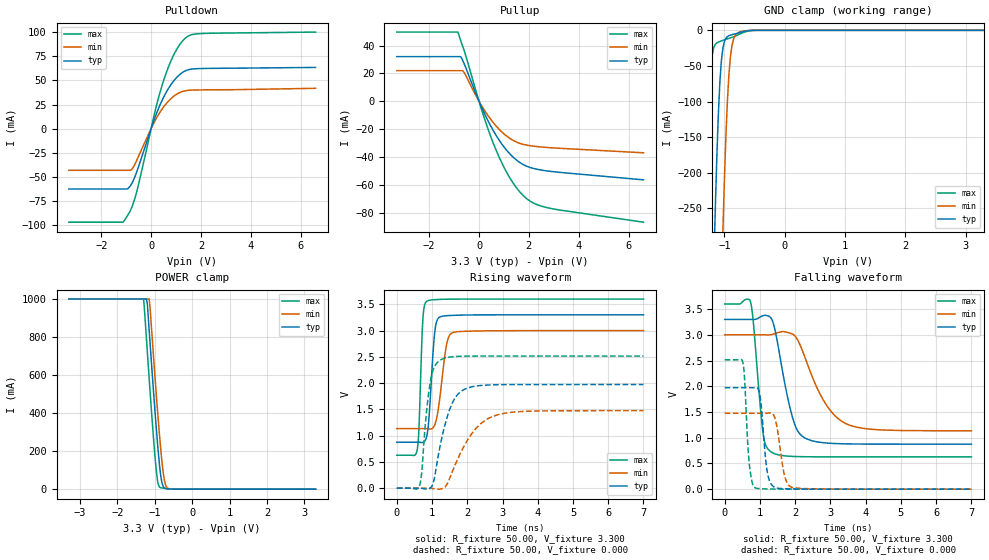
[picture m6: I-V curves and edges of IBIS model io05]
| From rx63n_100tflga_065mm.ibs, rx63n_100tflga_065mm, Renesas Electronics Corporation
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[Model]   io05
Model_type   I/O
Polarity   Non-Inverting
Enable   Active-High
Vinl  =   0.660V
Vinh  =   2.640V
Vmeas =   1.650V
Cref  =   30.00pF
| variable   typ   min   max
C_comp   3.770pF   3.770pF   3.770pF
| variable   typ   min   max
[Temperature Range]   45.000   105.000   -40.000
| variable   typ   min   max
[Voltage Range]   3.300V   3.000V   3.600V
| variable   typ   min   max
[Pullup Reference]   3.300V   3.000V   3.600V
| variable   typ   min   max
[Pulldown Reference]   0.000V   0.000V   0.000V
| variable   typ   min   max
[POWER Clamp Reference] 3.300V   3.000V   3.600V
| variable   typ   min   max
[GND Clamp Reference]   0.000V   0.000V   0.000V
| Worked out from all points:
|   slope of the pulldown table from 0 to 0.495 V, typ, clamps not added: 15.4 ohm
|   slope of the pullup table from 0 to 0.495 V, typ, clamps not added: 26.5 ohm
|   GND clamp passes 1 mA (typ) near -0.64 V on its own axis
|   POWER clamp passes 1 mA (typ) near -0.59 V on its own axis
|   rising waveform, R_fixture 50.00, V_fixture 3.300: 20-80 % time 140ps typ, 208ps min, 90.5ps max; typ from 0.875 V to 3.3 V
|   rising waveform, R_fixture 50.00, V_fixture 0.000: 20-80 % time 428ps typ, 745ps min, 217ps max; typ from 0 V to 1.97 V
|   falling waveform, R_fixture 50.00, V_fixture 3.300: 20-80 % time 432ps typ, 781ps min, 221ps max; typ from 3.3 V to 0.875 V
|   falling waveform, R_fixture 50.00, V_fixture 0.000: 20-80 % time 154ps typ, 198ps min, 122ps max; typ from 1.97 V to 0 V
[Pulldown]
| io05_strong Pulldown rx631_rx63n
| Thu Mar 22 17:15:49 2012
| voltage   I(typ)   I(min)   I(max)
-3.3V     -62.62mA   -43.25mA   -97.14mA
-1.15V    -62.62mA   -43.25mA   -97.14mA
-1.025V   -62.62mA   -43.25mA   -93.52mA
-800mV    -58.13mA   -42.94mA   -83.32mA
-600mV    -46.6mA    -34.2mA    -67.76mA
175mV     12.96mA    9.062mA    19.78mA
525mV     33.78mA    23.32mA    51.76mA
950mV     50.91mA    34.42mA    78.65mA
1.4V      60.32mA    39.47mA    94.53mA
1.7V      62.04mA    40.07mA    97.97mA
2.1V      62.47mA    40.25mA    98.84mA
6.6V      63.56mA    41.89mA    100.3mA
[Pullup]
| io05_strong Pullup rx631_rx63n
| Thu Mar 22 17:15:49 2012
| voltage   I(typ)   I(min)   I(max)
-3.3V     32.05mA    21.95mA    49.68mA
-850mV    32.05mA    21.95mA    49.68mA
-725mV    31.77mA    21.95mA    43.08mA
-625mV    28.07mA    21.43mA    37.88mA
175mV     -7.149mA   -5.281mA   -10.11mA
700mV     -24.99mA   -18.1mA    -35.76mA
1V        -32.82mA   -23.46mA   -47.4mA
1.325V    -39.44mA   -27.7mA    -57.61mA
1.95V     -46.99mA   -31.69mA   -70.56mA
2.3V      -48.81mA   -32.55mA   -74.14mA
2.9V      -50.5mA    -33.47mA   -77.15mA
6.6V      -56.53mA   -37.08mA   -86.96mA
[GND Clamp]
| io05_strong GNDClamp rx631_rx63n
| Thu Mar 22 17:15:49 2012
| voltage   I(typ)   I(min)   I(max)
-3.3V     -1A        -1A        -1A
-1.325V   -916.3mA   -1A        -321.6mA
-1.225V   -508.3mA   -1A        -56.05mA
-1.175V   -327.1mA   -831.8mA   -23.6mA
-1.15V    -246.5mA   -730.6mA   -19.51mA
-1.075V   -71.99mA   -445.9mA   -15.62mA
-1.025V   -24.89mA   -280.5mA   -14.09mA
-975mV    -11.12mA   -147.9mA   -12.65mA
-925mV    -7.484mA   -61.53mA   -11.26mA
-850mV    -5.559mA   -12.59mA   -9.146mA
-675mV    -1.555mA   -930uA     -2.738mA
3.3V      0A         0A         0A
[POWER Clamp]
| io05_strong PWRClamp rx631_rx63n
| Thu Mar 22 17:15:49 2012
| voltage   I(typ)   I(min)   I(max)
-3.3V     1A         1A         1A
-1.3V     1A         1A         1A
-1.225V   1A         1A         792.2mA
-1.2V     974.1mA    1A         720.1mA
-1.15V    831.4mA    1A         577.8mA
-975mV    355.2mA    535.2mA    125.1mA
-925mV    233.2mA    405.8mA    41.42mA
-875mV    126.6mA    283.8mA    11.35mA
-825mV    49.1mA     174.1mA    7.014mA
-750mV    7.224mA    53.11mA    4.912mA
-625mV    1.442mA    2.321mA    1.9mA
3.3V      0A         0A         0A
[Ramp]
dV/dt_r   1.184/427.74p  0.886/744.56p  1.509/216.62p
dV/dt_f   1.455/431.05p  1.119/780.77p  1.783/220.80p
R_load = 50.00ohm
[Rising Waveform]
| io05_strong Rising-High rx631_rx63n
| Thu Mar 22 17:15:49 2012
R_fixture = 50.00
V_fixture = 3.300
V_fixture_min = 3.000
V_fixture_max = 3.600
C_fixture = 0.00pF
| Time   V(typ)   V(min)   V(max)
0s        875mV      1.135V     628mV
575ps     876mV      1.135V     718mV
630ps     875mV      1.135V     1.161V
740ps     871mV      1.136V     3.21V
855ps     1.006V     1.133V     3.56V
1.075ns   2.955V     1.203V     3.588V
1.22ns    3.258V     1.714V     3.594V
1.415ns   3.283V     2.737V     3.597V
1.605ns   3.29V      2.967V     3.599V
7ns       3.3V       3V         3.6V
[Rising Waveform]
| io05_strong Rising-Low rx631_rx63n
| Thu Mar 22 17:15:49 2012
R_fixture = 50.00
V_fixture = 0.000
C_fixture = 0.00pF
| Time   V(typ)   V(min)   V(max)
0s        0V         0V         0V
655ps     0V         0V         69mV
950ps     3mV        -2mV       2.017V
1.065ns   184mV      -10mV      2.306V
1.25ns    871mV      -15mV      2.444V
1.485ns   1.469V     161mV      2.493V
1.715ns   1.774V     534mV      2.508V
2.205ns   1.94V      1.105V     2.514V
2.7ns     1.967V     1.36V      2.515V
7ns       1.974V     1.476V     2.515V
[Falling Waveform]
| io05_strong Falling-High rx631_rx63n
| Thu Mar 22 17:15:49 2012
R_fixture = 50.00
V_fixture = 3.300
V_fixture_min = 3.000
V_fixture_max = 3.600
C_fixture = 0.00pF
| Time   V(typ)   V(min)   V(max)
0s        3.3V       3V         3.6V
730ps     3.3V       3V         3.647V
815ps     3.299V     3V         3.228V
1.085ns   3.372V     3V         1.103V
1.325ns   3.315V     3.005V     721mV
1.915ns   1.417V     3.019V     637mV
2.255ns   1.003V     2.603V     631mV
2.855ns   899mV      1.669V     629mV
3.44ns    881mV      1.274V     628mV
7ns       875mV      1.135V     628mV
[Falling Waveform]
| io05_strong Falling-Low rx631_rx63n
| Thu Mar 22 17:15:49 2012
R_fixture = 50.00
V_fixture = 0.000
C_fixture = 0.00pF
| Time   V(typ)   V(min)   V(max)
0s        1.974V     1.476V     2.515V
515ps     1.974V     1.476V     2.465V
690ps     1.973V     1.476V     547mV
855ps     1.976V     1.476V     29mV
1.01ns    1.773V     1.476V     9mV
1.215ns   310mV      1.477V     4mV
1.405ns   40mV       1.419V     2mV
1.695ns   9mV        274mV      1mV
1.885ns   5mV        42mV       0V
7ns       0V         0V         0V
